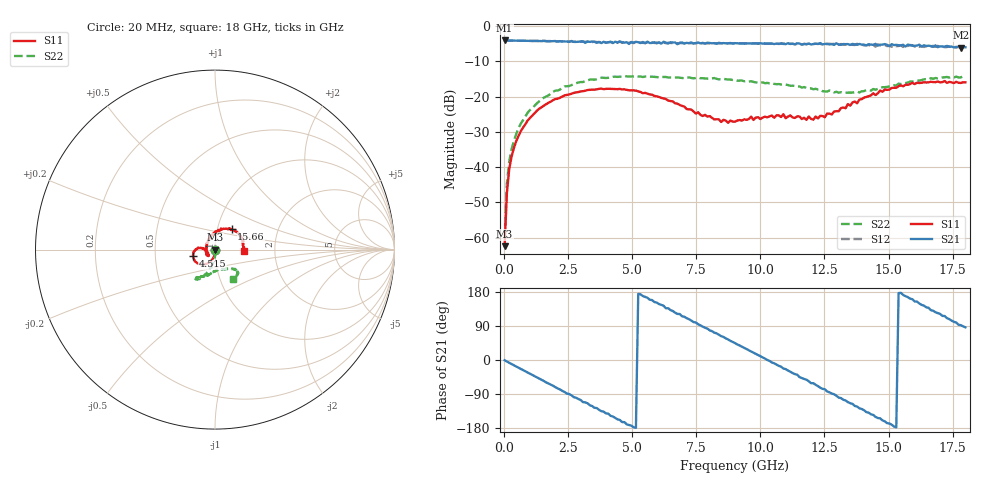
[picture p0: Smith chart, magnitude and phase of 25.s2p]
!Agilent Technologies,N5230A,US43500223,A.07.50.48
!Agilent N5230A: A.07.50.48
!Date: Sunday, January 31, 2016 11:26:33
!Correction: S11(Full 2 Port(1,2))
!S21(Full 2 Port(1,2))
!S12(Full 2 Port(1,2))
!S22(Full 2 Port(1,2))
!S2P File: Measurements: S11, S21, S12, S22:
# Hz S  dB  R 50
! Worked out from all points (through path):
!   201 points, 20 MHz to 18 GHz, reference 50 ohm
!   highest |S21| = -4.03 dB at 20 MHz (marker M1); lowest = -6.0 dB at 17.82 GHz (marker M2)
!   group delay of S21, straight-line fit = 97.6 ps
!   lowest |S11| = -62.5 dB at 20 MHz (marker M3), VSWR 1.00, Z = 50 - j0.0583 ohm
!   |S11| at or under -10 dB: start of sweep to end of sweep
!   |S22| runs from -60.1 to -14.1 dB; largest |S21 - S12| = 0.058
!   S11 on the Smith chart (normalised r, x): 20 MHz: 1.00, -0.00; 4.515 GHz: 0.78, -0.06; 15.66 GHz: 1.17, +0.28; 18 GHz: 1.38, -0.02
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2e7  -62.45 -50.6  -4.03 -0.8  -4.03 -0.9  -60.14 -99.5
1.099e8  -47.31 -77.4  -4.07 -4.1  -4.05 -4.1  -44.57 -79.7
1.998e8  -40.53 -82.9  -4.06 -7.3  -4.06 -7.4  -38.43 -83.8
3.796e8  -34.65 -89.8  -4.08 -13.9  -4.08 -14.0  -32.65 -87.8
6.493e8  -29.84 -94.3  -4.11 -23.5  -4.11 -23.6  -27.68 -90.5
1.818e9  -21.42 -117.8  -4.24 -65.0  -4.20 -65.8  -19.18 -105.0
3.0766e9  -18.44 -139.6  -4.27 -111.1  -4.37 -110.4  -15.83 -114.0
4.515e9  -17.77 -163.3  -4.35 -158.2  -4.28 -159.9  -14.33 -121.2
5.1443e9  -18.26 -172.7  -4.43 -179.0  -4.33 178.4  -14.09 -123.3
6.0433e9  -20.07 176.7  -4.55 147.7  -4.71 145.7  -14.48 -123.9
7.5716e9  -24.42 179.4  -4.61 94.2  -4.82 93.4  -14.58 -122.3
9.01e9  -27.08 -152.8  -4.79 44.7  -4.86 42.9  -15.24 -117.5
1.04484e10  -25.35 -140.2  -4.92 -6.5  -4.96 -8.0  -16.11 -108.5
1.20666e10  -26.53 170.1  -5.07 -61.1  -4.98 -65.1  -17.90 -98.6
1.28757e10  -24.23 130.2  -5.29 -90.3  -4.99 -94.6  -18.79 -85.9
1.35949e10  -21.62 103.6  -5.01 -115.8  -5.27 -121.1  -18.84 -74.0
1.44939e10  -19.52 77.9  -5.00 -150.1  -5.80 -151.8  -18.03 -57.7
1.50333e10  -18.00 66.3  -5.70 -167.6  -5.47 -172.5  -17.12 -49.8
1.56626e10  -16.61 51.2  -5.75 168.5  -5.43 167.0  -16.11 -46.0
1.68313e10  -15.87 22.1  -5.42 126.2  -5.86 123.9  -14.69 -45.2
1.78202e10  -16.10 1.7  -6.05 91.9  -6.04 87.4  -14.51 -54.2
1.8e10  -15.92 -2.3  -5.97 86.2  -6.02 81.2  -14.37 -59.1
